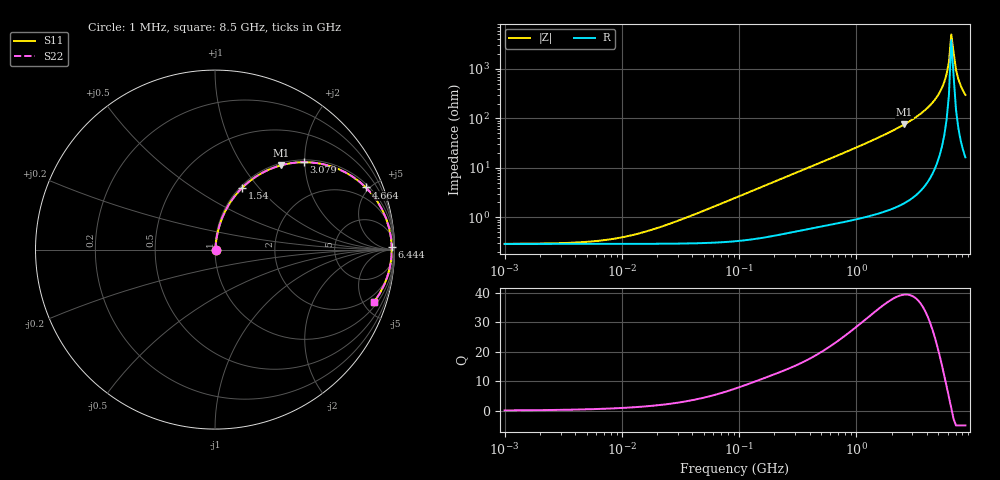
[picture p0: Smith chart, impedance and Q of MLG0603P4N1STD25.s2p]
! S-Parameter Data Generated by TDK Corporation
! Copyright(C) 2025 TDK Corporation.
! All Rights Reserved.
! TDK P/N: MLG0603P4N1STD25 (SMD / SMT Inductor (Coil))
! Property: L=4.1nH at 500MHz
! Size(LxWxT): 0.6x0.3x0.3mm
! Model Type: s2p (Touchstone File Format Version 1.0)
! Frequency: DC=Yes Start=1MHz Stop=8500MHz 198points Log-sweep
! Model Generated on Feb. 6, 2025
! Terms and conditions regarding TDK Simulation Models:
! 1)This simulation model is being provided solely for informational
!  purposes. Please refer to the specifications of the products in
!  terms of detailed characteristics of such products.
! 2)In no event shall TDK Corporation of any of its subsidiaries be
!  liable for any loss or damage arising, directly or indirectly,
!  from any information contained in this simulation model, including,
!  but not limited to loss or damages arising from any inaccuracies,
!  omissions or errors in connection with such information.
! 3)Any and all copyrights on this simulation model are owned by
!  TDK Corporation.  Duplication or redistribution of this simulation
!  model without prior written permission from TDK Corporation
!  is prohibited.
! 4)This simulation model is subject to any modification or change
!  without any prior notice.
! 5)Neither TDK Corporation nor any of its subsidiaries shall make any
!  warranty, express or implied, including but not limited to the
!  correctness, implied warranties of merchantability and fitness for
!  a particular purpose with respect to this simulation models.
! 6)The use of this simulation model shall be deemed to have consented
!  to the terms and conditions hereof.
! Port Assignments:
!  1 ---@@@--- 2
! Applicable Conditions:
!  Temperature = 25 degC
!  DC Bias Current = 0 A
!  Small Signal Operation
# Hz S MA R 50
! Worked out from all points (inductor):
!   197 points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, 1 MHz to 8.5 GHz, reference 50 ohm
!   read as one part in series: L = 4.23 nH near 33.39 MHz
!   highest Q = 39.3 at 2.56 GHz (marker M1), where L = 4.71 nH
!   self-resonance near 6.444 GHz
!   S11 on the Smith chart (normalised r, x): 1 MHz: 1.01, +0.00; 1.54 GHz: 1.02, +0.82; 3.079 GHz: 1.05, +1.98; 4.664 GHz: 1.19, +4.77; 6.444 GHz: open; 8.5 GHz: 1.33, -5.99
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1000000  0.002904 5.2  0.9971 -0.0  0.9971 -0.0  0.002904 5.2
4587603  0.003139 22.8  0.9971 -0.1  0.9971 -0.1  0.003139 22.8
1.005548e7  0.003939 42.5  0.9971 -0.2  0.9971 -0.2  0.003939 42.5
2.10461e7  0.0063 62.1  0.9971 -0.3  0.9971 -0.3  0.0063 62.1
9.219544e7  0.02457 81.0  0.9964 -1.4  0.9964 -1.4  0.02457 81.0
4.229561e8  0.1081 80.6  0.9882 -6.2  0.9882 -6.2  0.1081 80.6
9.270694e8  0.2313 74.5  0.9645 -13.4  0.9645 -13.4  0.2313 74.5
1.540426e9  0.376 66.3  0.9158 -22.1  0.9158 -22.1  0.376 66.3
1.940355e9  0.4662 60.7  0.8723 -27.8  0.8723 -27.8  0.4662 60.7
2.559585e9  0.5967 51.9  0.7874 -36.6  0.7874 -36.6  0.5967 51.9
3.07866e9  0.695 44.5  0.7012 -44.0  0.7012 -44.0  0.695 44.5
3.877948e9  0.8208 33.2  0.5473 -55.1  0.5473 -55.1  0.8208 33.2
4.664383e9  0.9094 22.4  0.3809 -65.3  0.3809 -65.3  0.9094 22.4
5.357206e9  0.9578 13.4  0.2322 -72.9  0.2322 -72.9  0.9578 13.4
5.610304e9  0.969 10.3  0.1791 -74.9  0.1791 -74.9  0.969 10.3
5.87536e9  0.9773 7.1  0.1249 -76.0  0.1249 -76.0  0.9773 7.1
6.152938e9  0.9826 3.9  0.07018 -73.7  0.07018 -73.7  0.9826 3.9
6.44363e9  0.9848 0.7  0.01969 -39.1  0.01969 -39.1  0.9848 0.7
7.066863e9  0.9796 -5.7  0.1004 75.4  0.1004 75.4  0.9796 -5.7
7.400733e9  0.9723 -8.9  0.155 75.3  0.155 75.3  0.9723 -8.9
7.750377e9  0.962 -12.0  0.2086 73.6  0.2086 73.6  0.962 -12.0
8.5e9  0.9335 -18.1  0.3114 68.8  0.3114 68.8  0.9335 -18.1
